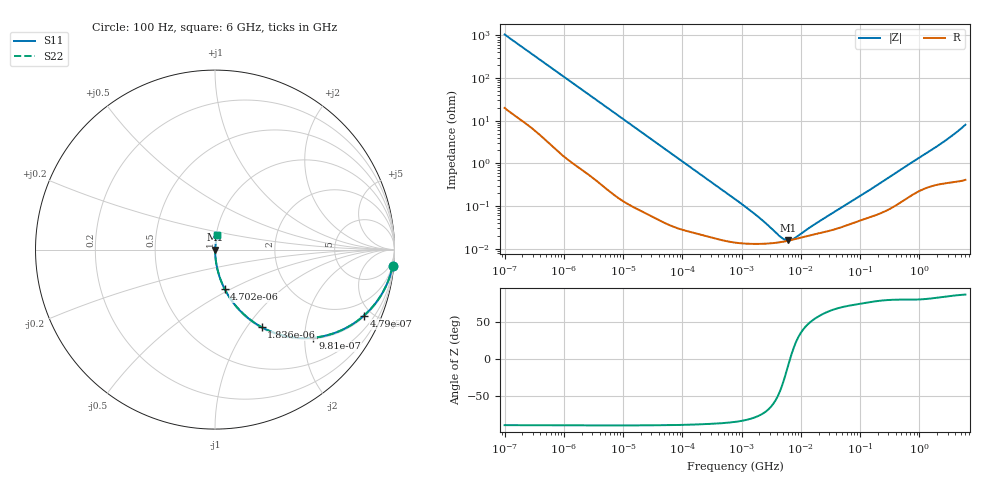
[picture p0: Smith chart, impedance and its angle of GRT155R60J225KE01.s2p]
!Murata Part Number: GRT155R60J225KE01
!These Parameters are Measured in Series Mode Connection
!Data Generated on Jun 19, 2026
!  o--ll--o
!Port1  Port2
!  o------o
!Operation Temp=25[degC], DC Bias Voltage=0[V]
!Freq. Start=100[Hz] Stop=6[GHz] 401[Steps]
# Hz S RI R 50
!Freq.(Hz) S11(Real) S11(Imag) S21(Real) S21(Imag) S12(Real) S12(Imag) S22(Real) S22(Imag)
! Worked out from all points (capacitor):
!   401 points, 100 Hz to 6 GHz, reference 50 ohm
!   read as one part in series: C = 1.51 uF near 109 Hz
!   lowest |Z| = 15.5 mohm at 6.075 MHz (marker M1)
!   series resonance near 6.573 MHz, so ESL is about 390 pH
!   S11 on the Smith chart (normalised r, x): 100 Hz: 1, -21; 479 Hz: 1.07, -4.46; 981 Hz: 1.03, -2.19; 1.836 kHz: 1.02, -1.18; 4.702 kHz: 1.01, -0.46; 6 GHz: 1.01, +0.16
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100  0.9893 -0.0941  0.0107 0.0941  0.0107 0.0941  0.9893 -0.0941
245  0.9458 -0.2174  0.0542 0.2174  0.0542 0.2174  0.9458 -0.2174
479  0.8288 -0.3686  0.1712 0.3686  0.1712 0.3686  0.8288 -0.3686
656  0.7251 -0.4391  0.2749 0.4391  0.2749 0.4391  0.7251 -0.4391
981  0.5454 -0.4912  0.4546 0.4912  0.4546 0.4912  0.5454 -0.4912
1342  0.3936 -0.482  0.6064 0.482  0.6064 0.482  0.3936 -0.482
1836  0.26 -0.4322  0.74 0.4322  0.74 0.4322  0.26 -0.4322
2008  0.2278 -0.4129  0.7722 0.4129  0.7722 0.4129  0.2278 -0.4129
3005  0.1186 -0.3169  0.8814 0.3169  0.8814 0.3169  0.1186 -0.3169
4702  0.0533 -0.2187  0.9467 0.2187  0.9467 0.2187  0.0533 -0.2187
12041  0.00929 -0.09  0.9907 0.09  0.9907 0.09  0.00929 -0.09
40335  0.00121 -0.0273  0.9988 0.0273  0.9988 0.0273  0.00121 -0.0273
774597  0.000141 -0.00145  0.9999 0.00145  0.9999 0.00145  0.000141 -0.00145
1983483  0.00013 -0.000518  0.9999 0.000518  0.9999 0.000518  0.00013 -0.000518
4643984  0.000143 -0.000117  0.9999 0.000117  0.9999 0.000117  0.000143 -0.000117
5311619  0.000148 -7.01e-05  0.9999 7.01e-05  0.9999 7.01e-05  0.000148 -7.01e-05
6075234  0.000153 -2.53e-05  0.9998 2.53e-05  0.9998 2.53e-05  0.000153 -2.53e-05
7947587  0.000167 5.93e-05  0.9998 -5.93e-05  0.9998 -5.93e-05  0.000167 5.93e-05
1.555665e7  0.000211 0.000269  0.9998 -0.000269  0.9998 -0.000269  0.000211 0.000269
3.124326e8  0.000865 0.00469  0.9991 -0.00469  0.9991 -0.00469  0.000865 0.00469
2.142435e9  0.0039 0.0264  0.9961 -0.0264  0.9961 -0.0264  0.0039 0.0264
6e9  0.0104 0.0792  0.9896 -0.0792  0.9896 -0.0792  0.0104 0.0792
